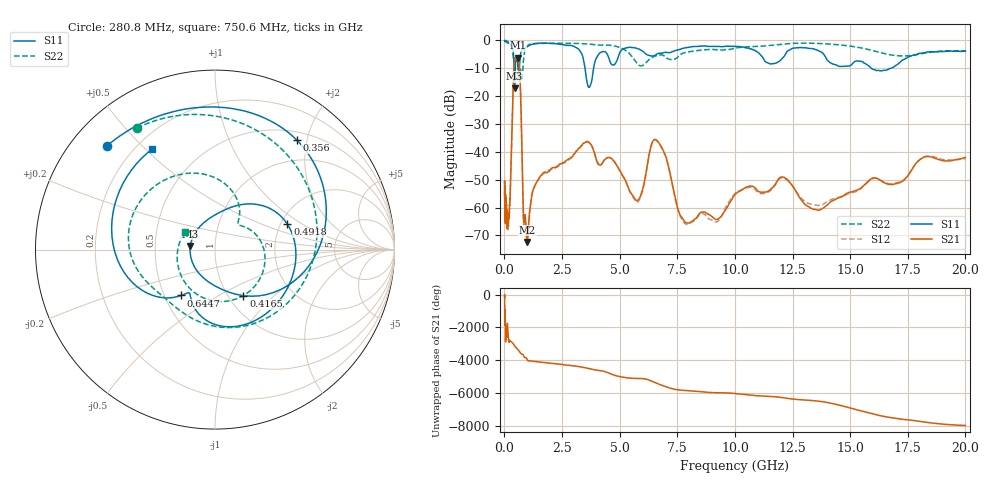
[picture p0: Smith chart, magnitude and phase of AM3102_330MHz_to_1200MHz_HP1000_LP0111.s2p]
! Date/Time: Tue, Sep 11, 2018 5:17 PM
! Network Analyzer: Agilent Technologies E8362B Rev: A.07.50.63
! Sweep from 0.010 to 20.000 GHz, 1601 Points, Sweep Type: LOG
! Power Supply: 4.949 V, 0.001 A
# Hz S DB R 50
!freq MagS11 AngS11 MagS21 AngS21 MagS12 AngS12 MagS22 AngS22
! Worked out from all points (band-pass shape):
!   1601 points, 10 MHz to 20 GHz, reference 50 ohm
!   highest |S21| = -6.20 dB at 586.3 MHz (marker M1); lowest = -72.4 dB at 988.7 MHz (marker M2)
!   |S21| within 3 dB of the highest: 413.5 MHz to 650.9 MHz (237.3 MHz wide, 44.6 % of centre)
!   lowest |S11| = -17.1 dB at 440.9 MHz (marker M3), VSWR 1.32, Z = 37.9 + j1.53 ohm
!   |S11| at or under -10 dB: 415.4 MHz to 469.5 MHz (54.14 MHz wide, 12.2 % of centre); 3.501 GHz to 3.87 GHz (369.6 MHz wide, 10 % of centre); 15.91 GHz to 16.76 GHz (851.5 MHz wide, 5.21 % of centre)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
!   |S22| runs from -14.5 to -0.2 dB; largest |S21 - S12| = 0.0092
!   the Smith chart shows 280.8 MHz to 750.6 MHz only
!   S11 on the Smith chart (normalised r, x): 280.8 MHz: 0.11, +0.40; 356 MHz: 0.63, +1.82; 416.5 MHz: 1.17, -0.66; 491.8 MHz: 2.18, +0.75; 644.7 MHz: 0.61, -0.35; 750.6 MHz: 0.26, +0.53
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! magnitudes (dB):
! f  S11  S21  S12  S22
! 10 MHz  0.0  -51.3  -51.7  -0.2
! 35.55 MHz  0.0  -63.1  -63.4  -0.4
! 126.4 MHz  -0.4  -63.3  -64.5  -0.9
! 217.2 MHz  -1.0  -60.3  -62.9  -1.3
! 280.8 MHz  -1.6  -47.3  -47.1  -1.9
! 356 MHz  -2.4  -24.0  -24.0  -4.2
! 416.5 MHz  -10.4  -8.8  -8.8  -7.7
! 440.9 MHz  -17.1  -6.6  -6.6  -8.2
! 447.2 MHz  -16.6  -6.4  -6.4  -8.1
! 491.8 MHz  -7.4  -6.4  -6.4  -6.2
! 586.3 MHz  -8.5  -6.2  -6.3  -9.9
! 644.7 MHz  -10.0  -8.5  -8.6  -13.9
! 750.6 MHz  -3.6  -34.7  -34.8  -14.2
! 833.3 MHz  -3.2  -64.3  -66.0  -6.6
! 988.7 MHz  -2.2  -72.4  -73.9  -2.0
! 1.59 GHz  -1.0  -48.5  -48.5  -1.0
! 3.107 GHz  -2.6  -39.8  -40.0  -1.1
! 3.617 GHz  -16.1  -36.4  -36.3  -1.3
! 5.652 GHz  -2.6  -56.8  -57.2  -7.1
! 6.58 GHz  -5.1  -35.7  -35.9  -5.5
! 7.995 GHz  -2.4  -65.6  -65.8  -4.1
! 20 GHz  -3.8  -42.0  -42.5  -3.7
